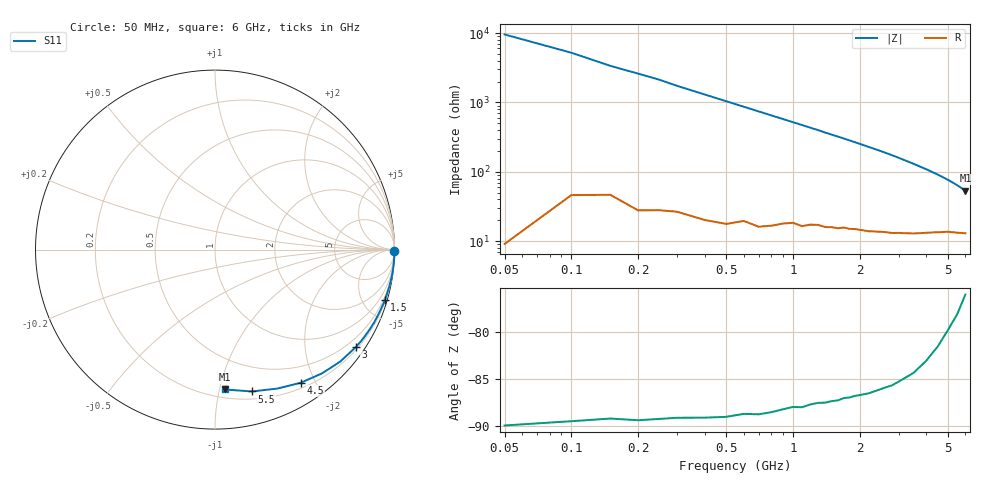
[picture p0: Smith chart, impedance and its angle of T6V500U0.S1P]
! SIEMENS Discrete & RF Semiconductors
! BAT62
! Si Schottky Diode in SOT143
! VR = 0.5 V
! S-Parameters:  February  1997
# GHz  S  MA  R  50
!  f  S11
! GHz  MAG  ANG
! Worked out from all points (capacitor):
!   34 points, 50 MHz to 6 GHz, reference 50 ohm
!   read as one part to ground: C = 315 fF near 50 MHz
!   lowest |Z| = 53.5 ohm at 6 GHz (marker M1)
!   S11 on the Smith chart (normalised r, x): 50 MHz: open; 1.5 GHz: 0.32, -6.84; 3 GHz: 0.26, -3.17; 4.5 GHz: 0.27, -1.80; 5.5 GHz: 0.27, -1.26; 6 GHz: 0.26, -1.04
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0.05  1 -0.6
0.1  0.9998 -1.1
0.15  0.9996 -1.7
0.25  0.9994 -2.7
0.3  0.9991 -3.3
0.4  0.9988 -4.4
0.7  0.9971 -7.7
0.8  0.9961 -8.8
1.1  0.9927 -12.1
1.3  0.9894 -14.3
1.4  0.9884 -15.5
1.5  0.9868 -16.6
1.6  0.9855 -17.7
1.7  0.9833 -18.8
1.8  0.982 -20.0
1.9  0.98 -21.1
2  0.9784 -22.3
2.2  0.9748 -24.7
2.4  0.9702 -27.1
2.6  0.9654 -29.5
2.8  0.9605 -32.1
3  0.9538 -34.8
3.5  0.936 -41.8
4  0.9115 -49.2
4.5  0.8824 -57.2
5  0.8488 -65.8
5.5  0.8167 -75.4
6  0.7812 -86.0
